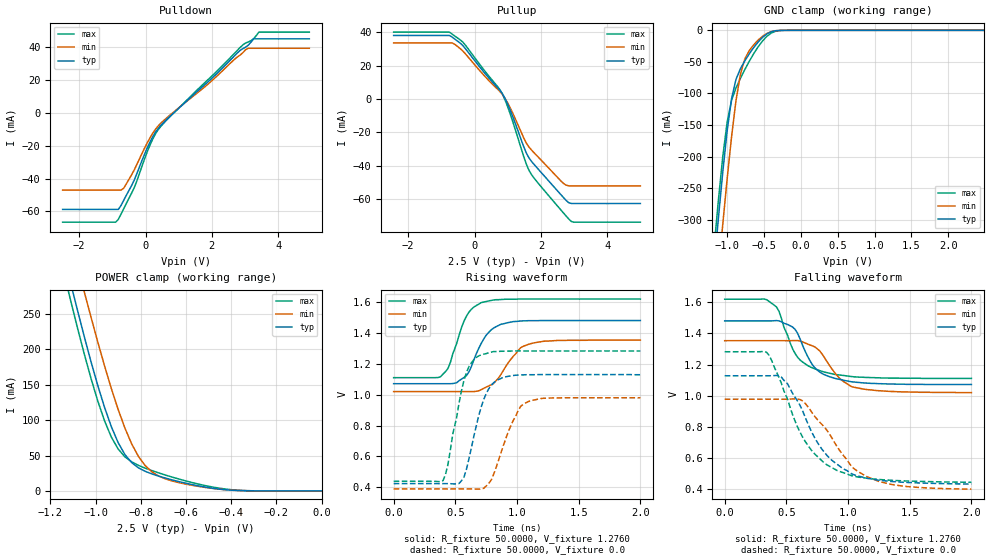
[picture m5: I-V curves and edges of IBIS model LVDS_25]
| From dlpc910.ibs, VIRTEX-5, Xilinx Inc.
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|   Model LVDS_25
[Model]  LVDS_25
Model_type I/O
Polarity   Non-Inverting
Enable   Active-Low
Vinl = 1.025
Vinh = 1.375
Vmeas =  1.2000V
Cref =   0.0F
Rref =   50.0000
Vref =   1.2000V
C_comp   6.0000pF   6.0000pF   6.0000pF
[Model Spec]
Vinl   1.025   0.125   2.025
Vinh   1.375   0.475   2.375
[Temperature Range]   25.0000   85.0000   0.0
[Voltage Range]   2.5000V   2.3750V   2.6250V
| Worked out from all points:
|   slope of the pulldown table from 0 to 0.375 V, typ, clamps not added: 26.5 ohm
|   slope of the pullup table from 0 to 0.375 V, typ, clamps not added: 40.6 ohm
|   GND clamp passes 1 mA (typ) near -0.36 V on its own axis
|   POWER clamp passes 1 mA (typ) near -0.40 V on its own axis
|   rising waveform, R_fixture 50.0000, V_fixture 1.2760: 20-80 % time 151ps typ, 183ps min, 136ps max; typ from 1.07 V to 1.48 V
|   rising waveform, R_fixture 50.0000, V_fixture 0.0: 20-80 % time 136ps typ, 169ps min, 126ps max; typ from 0.424 V to 1.13 V
|   falling waveform, R_fixture 50.0000, V_fixture 1.2760: 20-80 % time 176ps typ, 199ps min, 187ps max; typ from 1.48 V to 1.07 V
|   falling waveform, R_fixture 50.0000, V_fixture 0.0: 20-80 % time 320ps typ, 342ps min, 307ps max; typ from 1.13 V to 0.433 V
[Pulldown]
|Voltage   I(typ)   I(min)   I(max)
-2.5V     -58.82mA   -47.05mA   -66.6mA
-900mV    -58.82mA   -47.05mA   -66.6mA
-820mV    -58.82mA   -47.05mA   -64.85mA
-660mV    -53.37mA   -45.95mA   -58.5mA
-340mV    -40.92mA   -34.74mA   -45.56mA
140mV     -17.54mA   -15.04mA   -19.39mA
380mV     -9.514mA   -7.999mA   -10.28mA
2.86V     38.17mA    35.34mA    40mA
3.1V      41.29mA    39.39mA    43.24mA
3.26V     45.13mA    39.39mA    45.21mA
3.42V     45.13mA    39.39mA    49.24mA
4.94V     45.13mA    39.39mA    49.24mA
[Pullup]
|Voltage   I(typ)   I(min)   I(max)
-2.44V    38.01mA    33.58mA    40.03mA
-760mV    38.01mA    33.58mA    40.03mA
-600mV    35.9mA     32.75mA    37.71mA
-360mV    32.07mA    28.81mA    34.15mA
840mV     3.045mA    2.653mA    2.889mA
1.08V     -6.986mA   -5.606mA   -9.306mA
1.56V     -32.36mA   -26.41mA   -39.01mA
1.72V     -37.47mA   -30.68mA   -45.41mA
2.68V     -59.05mA   -50.6mA    -68.29mA
2.84V     -62.19mA   -52.05mA   -71.92mA
2.92V     -62.65mA   -52.11mA   -73.44mA
5V        -62.65mA   -52.11mA   -73.84mA
[GND_clamp]
|Voltage   I(typ)   I(min)   I(max)
-2.5V     -2.205A    -2.204A    -2.216A
-1.18V    -378.9mA   -462.7mA   -348.6mA
-1.12V    -300mA     -384.8mA   -271.2mA
-1.06V    -225.9mA   -308.6mA   -201.3mA
-1V       -159.8mA   -235.9mA   -145.6mA
-940mV    -108.6mA   -168.9mA   -111.1mA
-880mV    -77.83mA   -111.6mA   -91.37mA
-820mV    -60.88mA   -69.68mA   -76.15mA
-700mV    -37.32mA   -32.15mA   -49.15mA
-460mV    -5.634mA   -4.923mA   -9.418mA
-220mV    -16.94uA   -28.82uA   -46.49uA
2.48V     18.3nA     756.7nA    38.49nA
[POWER_clamp]
|Voltage   I(typ)   I(min)   I(max)
-2.49V    2.064A     2.03A      2.088A
-1.14V    332.1mA    390.5mA    308.4mA
-1.11V    293.9mA    354.2mA    269.3mA
-1.08V    255.9mA    317.9mA    230.9mA
-1.05V    218.6mA    281.8mA    194mA
-960mV    118.1mA    176.7mA    99.03mA
-900mV    68.31mA    115.3mA    59.3mA
-810mV    32.62mA    48.69mA    36.12mA
-750mV    23.96mA    26.81mA    28.67mA
-660mV    15.5mA     13.99mA    19.47mA
-480mV    3.661mA    3.472mA    5.36mA
0V        19.95nA    100nA      43.67nA
[Ramp]
| variable   typ   min   max
dV/dt_r  0.4231/0.1360n   0.3541/0.1690n   0.5065/0.1160n
dV/dt_f  0.1662/85.6439p   0.1362/0.1020n   0.2046/76.2034p
R_load = 50.0000
[Rising Waveform]
R_fixture= 50.0000
V_fixture= 1.2760
V_fixture_min= 1.1870
V_fixture_max= 1.3650
|time   V(typ)   V(min)   V(max)
0s        1.071V     1.02V      1.11V
380ps     1.071V     1.02V      1.116V
440ps     1.071V     1.02V      1.169V
590ps     1.123V     1.02V      1.508V
710ps     1.332V     1.032V     1.596V
790ps     1.419V     1.064V     1.61V
870ps     1.456V     1.131V     1.616V
1.03ns    1.477V     1.304V     1.619V
1.11ns    1.479V     1.33V      1.619V
2ns       1.48V      1.353V     1.619V
[Rising Waveform]
R_fixture= 50.0000
V_fixture= 0.0
|time   V(typ)   V(min)   V(max)
0s        423.9mV    389.4mV    438.9mV
400ps     423.9mV    389.4mV    443.1mV
440ps     423.9mV    389.4mV    547.3mV
570ps     465.6mV    389.4mV    1.093V
610ps     583.7mV    389.4mV    1.181V
690ps     865.3mV    388mV      1.251V
810ps     1.077V     482.9mV    1.279V
930ps     1.119V     761.5mV    1.282V
1.05ns    1.128V     937.3mV    1.283V
2ns       1.129V     979.5mV    1.283V
[Falling Waveform]
R_fixture= 50.0000
V_fixture= 1.2760
V_fixture_min= 1.1870
V_fixture_max= 1.3650
|time   V(typ)   V(min)   V(max)
0s        1.48V      1.353V     1.619V
320ps     1.48V      1.353V     1.62V
400ps     1.481V     1.353V     1.582V
440ps     1.48V      1.353V     1.542V
590ps     1.402V     1.354V     1.248V
690ps     1.226V     1.326V     1.186V
770ps     1.152V     1.288V     1.161V
910ps     1.108V     1.13V      1.135V
1.03ns    1.089V     1.058V     1.123V
2ns       1.072V     1.02V      1.111V
[Falling Waveform]
R_fixture= 50.0000
V_fixture= 0.0
|time   V(typ)   V(min)   V(max)
0s        1.128V     977.7mV    1.282V
340ps     1.128V     977.7mV    1.278V
460ps     1.119V     977.6mV    1.078V
510ps     1.076V     977.7mV    977mV
630ps     905.8mV    967.2mV    736.4mV
770ps     677.6mV    830.5mV    596.2mV
910ps     561.1mV    674.7mV    520.8mV
1.03ns    498.5mV    544.1mV    486.7mV
1.25ns    458mV      450.2mV    462.9mV
2ns       432.9mV    400.5mV    444.5mV
